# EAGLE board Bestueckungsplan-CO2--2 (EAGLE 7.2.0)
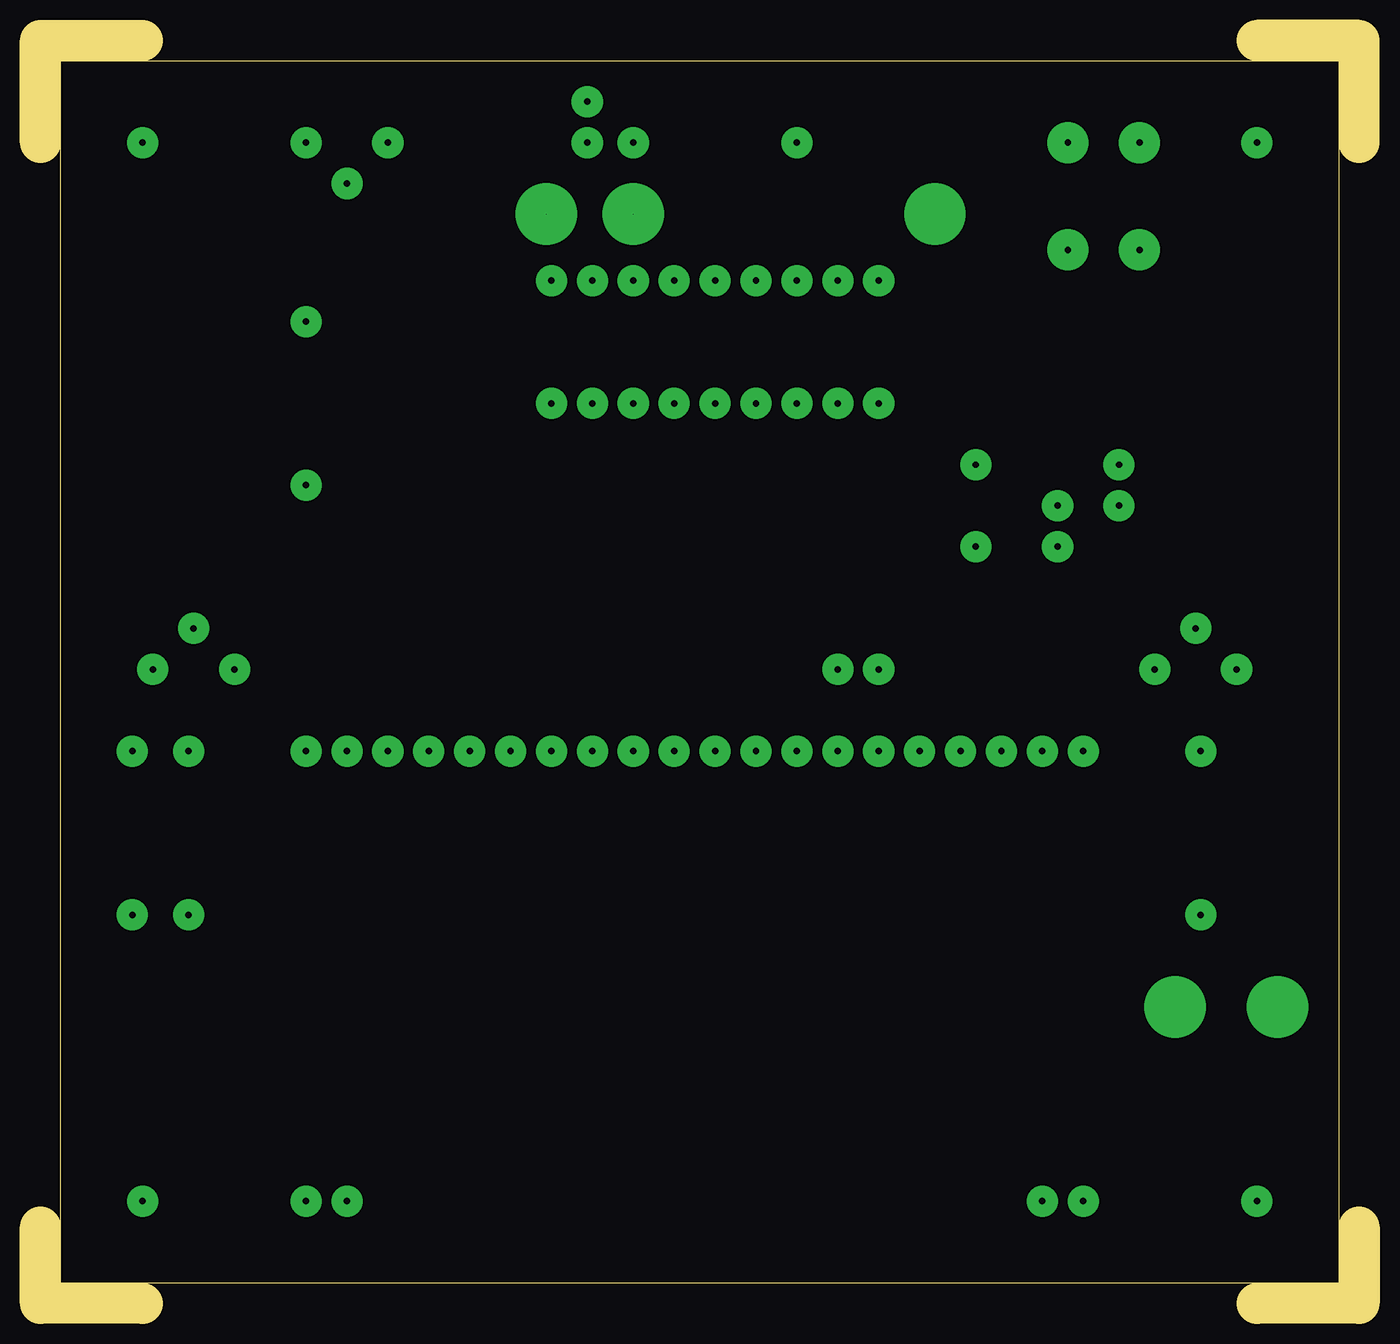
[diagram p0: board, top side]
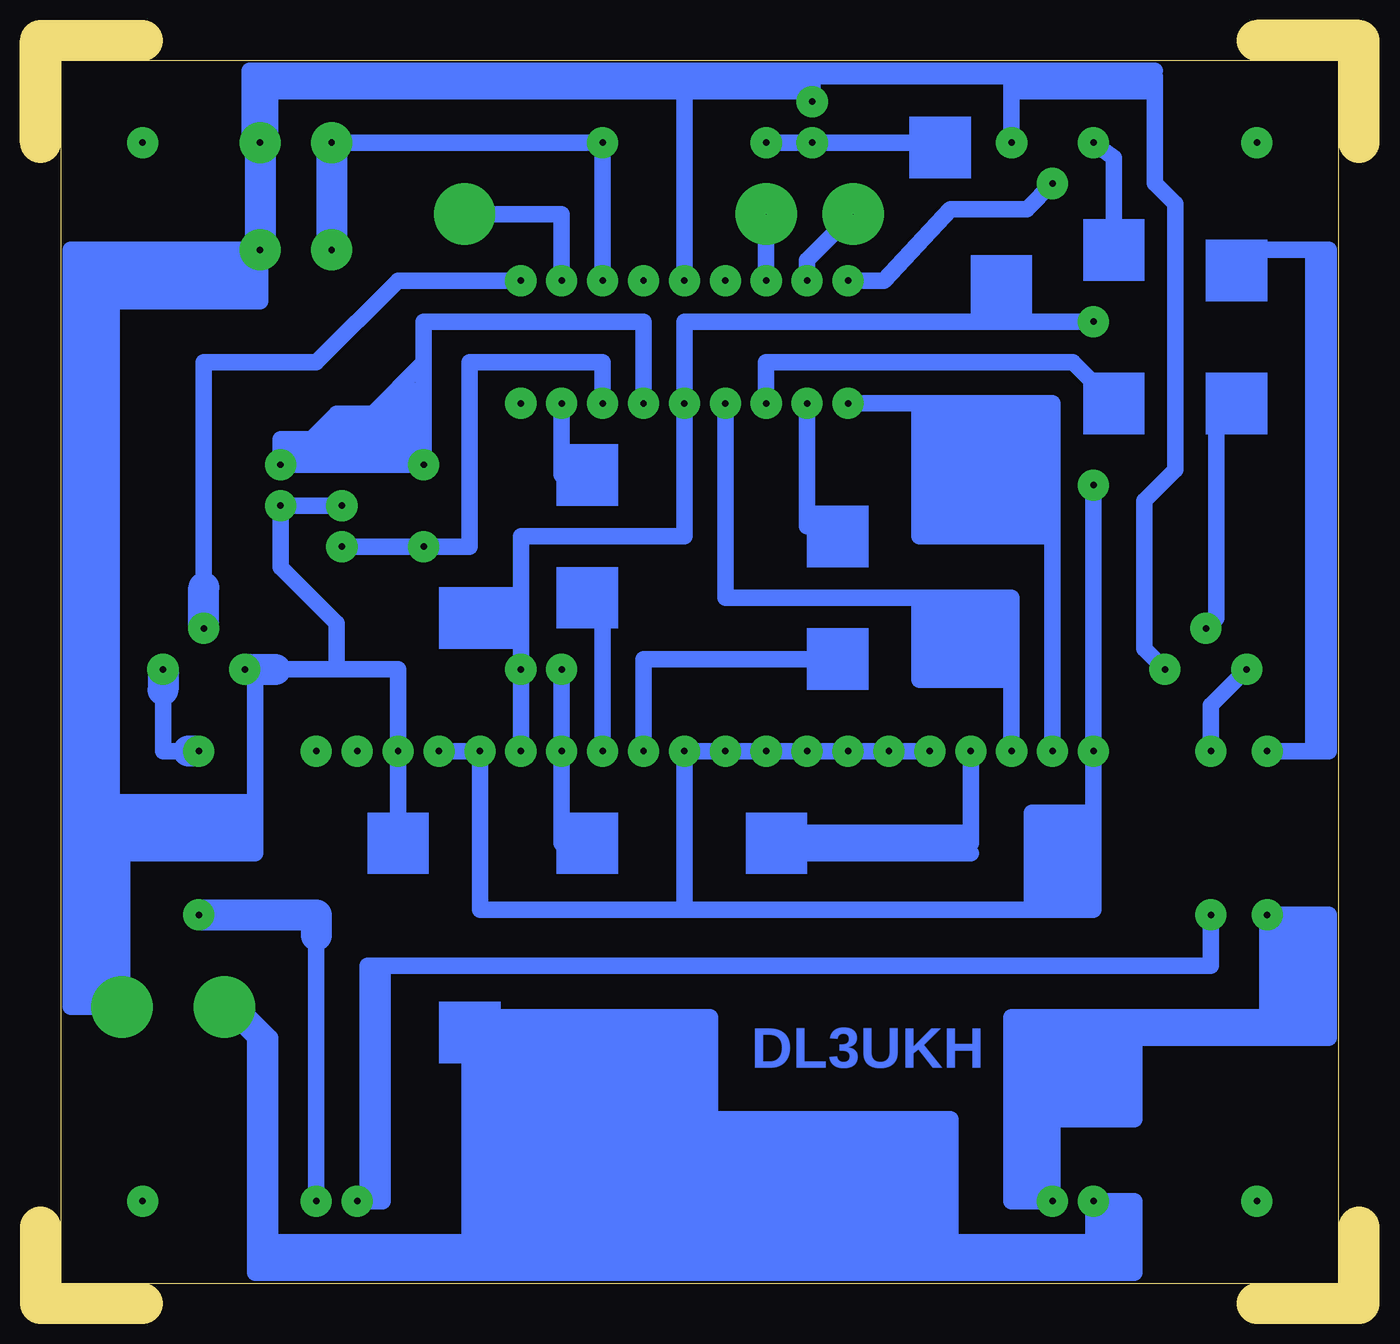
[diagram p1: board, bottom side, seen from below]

Size 81.91 x 78.42 mm. Coordinates in mm from the lower left corner, seen from the top.
Outline: 81.91,72.07 81.91,78.42 75.56,78.42
Outline: 81.91,4.76 81.91,0 75.56,0
Outline: 6.35,0 0,0 0,4.76
Outline: 0,72.07 0,78.42 6.35,78.42
Outline: 80.64,77.15 80.64,1.27 1.27,1.27 1.27,77.15 80.64,77.15
Copper layers (1*16): Top 0.035mm / dielectric 1.5mm / Bottom 0.035mm
Design rules "default": minimum track width 10mil, minimum drill 24mil, track to track 8mil, track to pad 8mil, pad to pad 8mil, via to via 8mil, smd to smd 8mil, copper to edge 40mil, drill to drill 8mil, minimum pad ring 10mil, minimum via ring 8mil, stop-mask expansion 4mil, vias tented up to drill 0mil, thermal gap 10mil

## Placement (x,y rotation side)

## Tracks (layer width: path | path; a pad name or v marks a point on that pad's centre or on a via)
S$1  (via drill 0.4 pad 1.93)
  Bottom 1.016: v52.07,34.29 v52.07,39.37 52.07,42.55 | 52.07,42.55 52.07,47.62 41.91,47.62 v41.91,55.88 41.91,60.96 16.51,60.96 | 52.07,42.55 55.25,42.55
S$2  (via drill 0.4 pad 1.93)
  other vias: 31.75,34.29
S$3  (via drill 0.4 pad 1.93)
  Bottom 1.016: v36.83,55.88 36.83,58.42 17.78,58.42 15.24,55.88
S$4  (via drill 0.4 pad 1.93)
  Bottom 1.016: v34.29,55.88 34.29,48.26 32.38,48.26
S$5  (via drill 0.4 pad 1.93)
  Bottom 1.016: v49.53,55.88 49.53,51.44 47.94,51.44
S$6  (via drill 0.01 pad 3.81, 0.4 pad 1.93, 0.4 pad 2.54)
  Bottom 1.016: v12.06,39.37 13.33,40.64 13.33,49.85 11.43,51.75 11.43,68.26 12.7,69.53 12.7,75.25 | 12.7,75.25 12.7,76.2 21.59,76.2 | 77.47,65.41 v68.26,65.41 68.26,62.23 77.47,62.23 | 77.47,65.41 77.47,62.23 | 77.47,62.23 77.47,31.11 | 77.47,31.11 76.83,31.11 | 76.83,31.11 68.58,31.11 | v68.26,72.07 68.26,75.25 | 68.26,75.25 68.26,76.2 | 68.26,76.2 67.94,76.2 | 67.94,76.2 41.91,76.2 | 41.91,76.2 41.91,75.25 | 41.91,75.25 v41.91,63.5 | 41.91,76.2 33.97,76.2 | 33.97,76.2 21.59,76.2 | v21.59,72.07 21.59,76.2 | 68.58,31.11 68.58,38.74 v69.21,39.37 | v63.18,49.53 v66.99,49.53 66.99,45.72 63.5,42.23 63.5,39.37 | 67.31,39.37 63.5,39.37 | 63.5,39.37 59.69,39.37 v59.69,34.29 59.69,28.89 | 33.97,76.2 33.97,75.25 | 33.97,75.25 v33.97,74.61 | 76.83,31.11 v76.83,18.41 80.01,18.41 80.01,31.11 | 77.47,31.11 80.01,31.11 | 68.58,31.11 68.58,27.94 77.15,27.94 | 77.47,65.41 80.01,65.41 80.01,31.11 | 68.26,76.2 68.26,76.52 | 68.26,76.52 67.94,76.52 | 67.94,76.52 12.7,76.52 | 41.91,75.25 68.26,75.25 | 41.91,75.25 33.97,75.25 | 12.7,75.25 21.27,75.25 | 67.94,76.2 67.94,76.52 | 68.26,76.52 68.9,76.52 68.9,72.07
  Bottom 1.93: v68.26,72.07 v68.26,65.41 | v69.21,39.37 67.31,39.37
S$7  (via drill 0.4 pad 1.93)
  Bottom 1.016: v49.53,63.5 49.53,67.63 55.56,67.63
S$8  (via drill 0.4 pad 1.93)
  other vias: 6.35,6.35
S$9  (via drill 0.4 pad 1.93)
  other vias: 6.35,72.07
S$10  (via drill 0.4 pad 1.93)
  Bottom 1.016: v36.83,72.07 26.04,72.07
S$11  (via drill 0.4 pad 1.93)
  other vias: 34.29,34.29
S$12  (via drill 0.4 pad 1.93)
  Bottom 1.016: 60.64,20.95 60.33,20.95 9.21,20.95 v9.21,24.13 | 60.64,20.95 60.64,6.35 61.6,6.35 | 61.6,6.35 v62.23,6.35 | 61.6,6.35 61.6,20.95 60.64,20.95
S$13  (via drill 0.4 pad 1.93)
  other vias: 16.51,60.96
S$14  (via drill 0.4 pad 1.93)
  Bottom 1.016: v44.45,34.29 44.45,40.01 32.38,40.01
S$15  (via drill 0.4 pad 1.93)
  Bottom 1.016: v24.13,34.29 24.13,29.21 | 24.13,29.21 24.13,28.57 35.24,28.57 | 24.13,29.21 34.93,29.21
S$16  (via drill 0.4 pad 1.93)
  Bottom 1.016: v16.51,72.07 15.24,71.12 15.24,65.41
S$17  (via drill 0.4 pad 1.93)
  Bottom 1.016: v9.53,41.91 8.89,42.55 8.89,55.25
S$18  (via drill 0.4 pad 1.93)
  Bottom 1.016: 13.65,16.51 6.03,16.51 5.71,16.51 | 19.05,17.78 21.59,17.78 21.59,6.35 v19.05,6.35 19.05,11.43 | 19.05,17.78 13.97,17.78 | 13.97,17.78 5.71,17.78 | 5.71,17.78 v5.71,24.13 1.91,24.13 1.91,16.51 5.71,16.51 | 19.05,11.43 19.05,17.78 | 13.97,17.14 13.97,11.43 19.05,11.43 | 13.97,17.14 13.97,17.78 | 5.71,16.51 5.71,17.14 | 5.71,17.78 5.71,17.14 | 5.71,17.14 13.97,17.14
S$19  (via drill 0.4 pad 1.93)
  Bottom 1.016: v64.77,6.35 64.77,22.86
  Bottom 1.93: v72.07,24.13 64.77,24.13 64.77,22.86
S$20  (via drill 0.4 pad 1.93)
  Bottom 1.016: v46.99,55.88 46.99,58.42 55.25,58.42 55.25,46.99 v58.1,46.99 v63.18,46.99
S$21  (via drill 0.4 pad 1.93)
  Bottom 1.016: v36.83,63.5 36.83,67.31
S$22  (via drill 0.4 pad 1.93)
  other vias: 52.07,55.88
S$23  (via drill 0.4 pad 1.93)
  Bottom 1.016: v16.51,50.8 v16.51,34.29 16.51,30.48 | 16.51,30.48 16.51,24.45 20.32,24.45 | 20.32,24.45 41.91,24.45 | v26.67,34.29 v29.21,34.29 v36.83,34.29 v41.91,34.29 41.91,24.45 | v57.15,34.29 v54.61,34.29 54.61,24.45 41.91,24.45 | 16.51,30.48 20.32,30.48 20.32,24.45
S$24  (via drill 0.4 pad 1.93)
  Bottom 1.016: v46.99,34.29 46.99,42.86
S$25  (via drill 0.4 pad 1.93)
  other vias: 62.23,34.29
S$26  (via drill 0.4 pad 1.93)
  other vias: 64.77,34.29
S$27  (via drill 0.4 pad 1.93)
  Bottom 1.016: v5.71,34.29 3.49,34.29 2.86,34.29 | 2.86,34.29 2.86,65.41 | 2.86,65.41 8.89,65.41 | 2.86,65.41 1.91,65.41 1.91,34.29 2.86,34.29
S$28  (via drill 0.01 pad 3.81, 0.4 pad 1.93)
  Bottom 1.016: 54.93,17.78 40.32,17.78 40.32,11.43 | 16.51,3.81 v16.51,6.35 13.97,6.35 13.97,2.54 | 16.51,3.81 16.51,2.54 | 16.51,2.54 55.25,2.54 | 55.25,2.54 55.25,11.43 | 55.25,11.43 55.25,16.83 | 55.25,2.54 68.58,2.54 | 68.58,2.54 68.58,3.81 | 68.58,3.81 68.58,16.51 | 68.58,16.51 v70.48,18.41 | 13.97,2.54 16.51,2.54 | 16.51,3.81 68.58,3.81 | 13.97,2.54 13.97,1.91 68.58,1.91 68.58,2.54 | 25.4,3.17 25.4,11.43 40.32,11.43 | 40.32,11.43 55.25,11.43 | 68.58,16.51 67.63,16.51 | 67.63,16.51 67.63,3.17 | 67.63,16.51 70.17,19.05
S$29  (via drill 0.4 pad 1.93)
  other vias: 75.56,6.35
S$30  (via drill 0.4 pad 1.93)
  Bottom 1.016: 71.75,44.45 71.75,58.42 64.77,58.42 59.69,63.5 v52.07,63.5
  Bottom 1.93: v71.75,41.91 71.75,44.45
S$31  (via drill 0.4 pad 1.93)
  Bottom 1.016: v31.75,63.5 29.53,63.5 25.4,67.94 20.64,67.94 v19.05,69.53
S$32  (via drill 0.4 pad 1.93)
  other vias: 39.37,63.5
S$33  (via drill 0.4 pad 1.93)
  Bottom 1.016: 72.71,34.29 74.3,34.29 74.3,38.1
  Bottom 1.93: v74.3,39.37 74.3,38.1 | v72.07,34.29 72.71,34.29
S$34  (via drill 0.4 pad 1.93)
  other vias: 75.56,72.07
S$35  (via drill 0.4 pad 1.93)
  Bottom 1.016: v49.53,39.37 v49.53,34.29 49.53,28.57
S$36
  Bottom 1.016: 24.13,27.94 34.29,27.94
S$37  (via drill 0.01 pad 3.81)
  other vias: 36.83,67.63
S$38  (via drill 0.01 pad 3.81, 0.4 pad 1.93)
  Bottom 1.016: v19.05,34.29 19.05,47.62 | 19.05,47.62 19.05,55.88 27.3,55.88 | 27.3,55.88 v31.75,55.88 | v34.29,63.5 34.29,64.77 v31.43,67.63 31.11,67.94 | 19.05,47.62 27.3,47.62 27.3,55.88
S$39  (via drill 0.01 pad 3.81)
  other vias: 55.56,67.63
S$40  (via drill 0.01 pad 3.81)
  other vias: 90.49,41.91
S$41  (via drill 0.4 pad 1.93)
  other vias: 44.45,63.5
S$42  (via drill 0.4 pad 1.93)
  Bottom 1.016: v6.98,39.37 9.21,37.15 v9.21,34.29
S$43
  Bottom 1.016: 67.63,72.07 67.63,75.56
S$44  (via drill 0.4 pad 1.93)
  Bottom 1.016: v21.59,34.29 21.59,38.74 | 21.59,38.74 21.59,43.82 27.3,43.82 | 27.3,43.82 39.37,43.82 v39.37,55.88 | 21.59,38.74 27.3,38.74 27.3,43.82
S$45  (via drill 0.4 pad 1.93, 0.4 pad 2.54)
  Bottom 1.016: v46.99,63.5 v46.99,72.07 v63.82,72.07
  Bottom 1.93: v63.82,72.07 v63.82,65.41
S$46  (via drill 0.4 pad 1.93)
  other vias: 33.97,72.07
S$48  (via drill 0.4 pad 1.93)
  other vias: 39.37,34.29
S$57  (via drill 0.4 pad 1.93)
  Bottom 1.016: v44.45,55.88 44.45,60.96 58.1,60.96 58.1,58.42 | 58.1,58.42 v58.1,52.07 v66.99,52.07 66.99,53.66 65.09,53.66 63.5,55.25 61.28,55.25 58.1,58.42
(copper drawn outside any net)
  shapes: Bottom area x36

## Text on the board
Bottom: DL3UKH
Pads: AUF BESTÜCKUNGS-SEITE GESEHEN
Vias: 1 | 2 | 3 | 1 | 2 | 3 | +5V | -
Dimension: 1 stck. Taster 1,0mm
tOrigins: PIC16F1827 | 2N7000 | 1 | Links oben ist | immer PIN 1 | D | 47n | 10K | S | D | Taster | Br. | Br. | BOHRUNGEN: | G | alles 0.8mm | 1 | 4Stck. Befestigungsbohr... 3,5mm | Br. | 10K | Quarz | Leiterplatte: | 15p | 1,5mm dick | Cevausit | Br. | 15p | Br. | Für Anschlüsse | D | D | Siehe Stromlaufplan | 47n | Auch die 5,0Volt | 680 | 680 | 680 | 40 | 35 | 30 | 25 | 21 | Auf Leiterzugseite anlöten | Br. | Br. | Für die 8stck. Brücken | Br. | Br. | Die Lötinseln | Vergleiche mit Stromlaufplan | 19 | Auf Leiterzugseite anlöten | 2 | 1 | LCD-Display | 20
